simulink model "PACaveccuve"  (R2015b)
settings: Solver=ode15s  StartTime=0.0  StopTime=6000  RelTol=1e-3
libraries: fl_lib x9, nesl_utility x6

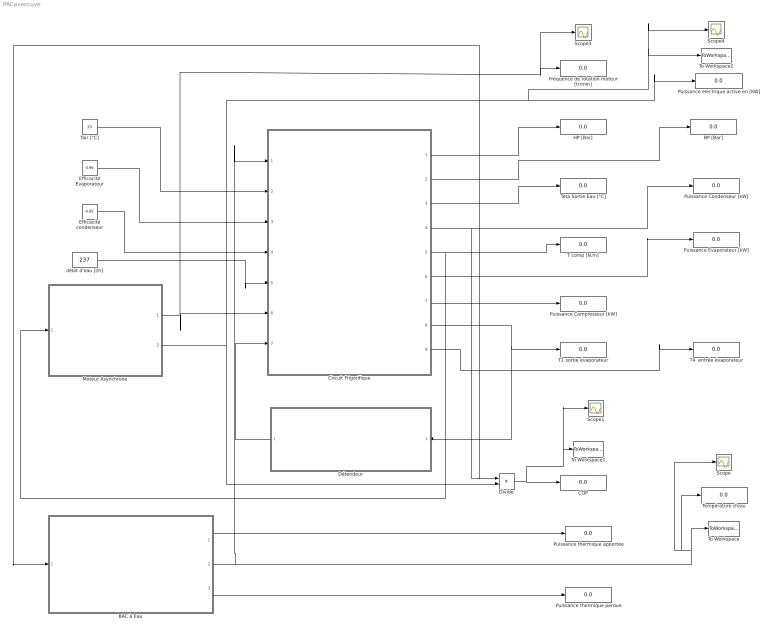
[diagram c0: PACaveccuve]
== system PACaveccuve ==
  BAC à Eau : Subsystem
  BP [Bar] : Display
  COP : Display
  Circuit Frigorifique : Subsystem
  Divide : Product  Inputs=*/
  Détendeur : Subsystem
  Efficacité Evaporateur : Constant  Value=0.99
  Efficacité condenseur : Constant  Value=0.95
  Fréquence de rotation moteur [tr/min] : Display
  HP [Bar] : Display
  Moteur Asynchrone : Subsystem
  Puissance Compresseur [kW] : Display
  Puissance Condenseur [kW] : Display
  Puissance Evaporateur [kW] : Display
  Puissance electrique active en [KW] : Display
  Puissance thermique apportée : Display
  Puissance thermique perdue : Display
  Scope{,1,3..4} (4 alike) : Scope
  T comp [N.m] : Display
  T1 sortie évaporateur : Display
  T4  entrée évaporateur : Display
  Tair [°C] : Constant  Value=23
  Température d'eau : Display
  Teta Sortie Eau [°C] : Display
  To Workspace : ToWorkspace  VariableName=Ts  SaveFormat=Timeseries  SampleTime=-1
  To Workspace1 : ToWorkspace  VariableName=COP  SaveFormat=Timeseries  SampleTime=-1
  To Workspace2 : ToWorkspace  VariableName=Pelec  SaveFormat=Timeseries  SampleTime=-1
  débit d'eau [l/h] : Constant  Value=237
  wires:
  Efficacité Evaporateur/1 -> Circuit Frigorifique/3(Eff Evapo)
  débit d'eau [l/h]/1 -> Circuit Frigorifique/5(Qv eau [l/h])
  Circuit Frigorifique/1(HP [bar]) -> HP [Bar]/1
  Circuit Frigorifique/2(BP [bar]) -> BP [Bar]/1
  Circuit Frigorifique/3(Tse [°C]) -> Teta Sortie Eau [°C]/1
  Circuit Frigorifique/5(Tm [N.m]) -> Moteur Asynchrone/1(Tm [N.m]), T comp [N.m]/1
  Circuit Frigorifique/9(T4 [°C]) -> T4  entrée évaporateur/1
  Circuit Frigorifique/8(T1 [°C]) -> Détendeur/1(T1), T1 sortie évaporateur/1
  Circuit Frigorifique/6(Pevapo [kW]) -> Puissance Evaporateur [kW]/1
  Divide/1 -> To Workspace1/1, Scope1/1, COP/1
  Circuit Frigorifique/7(Pcomp [kW]) -> Puissance Compresseur [kW]/1
  Efficacité condenseur/1 -> Circuit Frigorifique/4(effc)
  Détendeur/1(BP [Bar]) -> Circuit Frigorifique/7(BP[Bar])
  Moteur Asynchrone/2(Puissance Electrique active [W]) -> Scope4/1, To Workspace2/1, Puissance electrique active en [KW]/1, Divide/2
  Moteur Asynchrone/1(N [tr/min]) -> Scope3/1, Fréquence de rotation moteur [tr/min]/1, Circuit Frigorifique/6(N [tr/min])
  Tair [°C]/1 -> Circuit Frigorifique/2(Tair [°C])
  Circuit Frigorifique/4(Pcond [kW]) -> BAC à Eau/1(" Puissance Condenseur [kW]"), Divide/1, Puissance Condenseur [kW]/1
  BAC à Eau/2(Température du BAC [°C]) -> Scope/1, Température d'eau/1, To Workspace/1, Circuit Frigorifique/1(Tee [°C])
  BAC à Eau/1(Puissance Condenseur [W]) -> Puissance thermique apportée/1
  BAC à Eau/3(Puissance thermique perdue [W]) -> Puissance thermique perdue/1

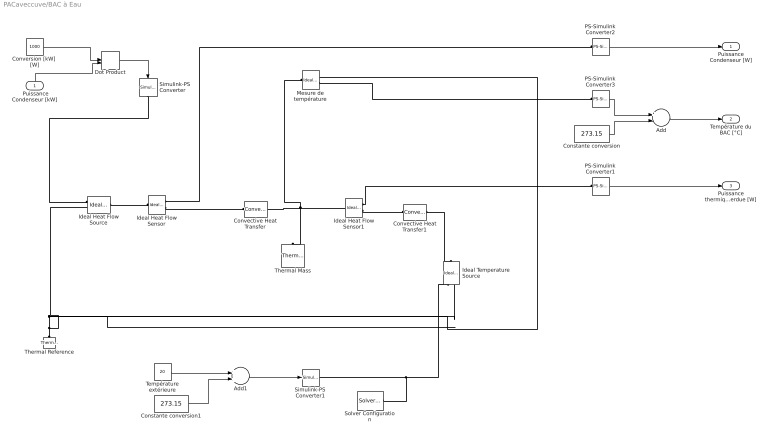
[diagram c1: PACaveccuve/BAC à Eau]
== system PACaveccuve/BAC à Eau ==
  " Puissance Condenseur [kW]" : Inport
  Add : Sum  Inputs=+-
  Add1 : Sum
  Constante conversion : Constant  Value=273.15
  Constante conversion1 : Constant  Value=273.15
  Convective Heat Transfer : fl_lib/Thermal/Thermal Elements/Convective Heat Transfer  area=1 m^2  heat_tr_coeff=1000000 W/(m^2 * K)  Q_specify=off  Q_priority=None  Q=0 J/s  T_specify=off  T_priority=None  T=0 K
  Convective Heat Transfer1 : fl_lib/Thermal/Thermal Elements/Convective Heat Transfer  area=1 m^2  heat_tr_coeff=10.3 W/(m^2 * K)  Q_specify=off  Q_priority=None  Q=0 J/s  T_specify=off  T_priority=None  T=0 K
  Conversion [kW]  [W] : Constant  Value=1000
  Dot Product : DotProduct
  Ideal Heat Flow Sensor : fl_lib/Thermal/Thermal Sensors/Ideal Heat Flow Sensor
  Ideal Heat Flow Sensor1 : fl_lib/Thermal/Thermal Sensors/Ideal Heat Flow Sensor
  Ideal Heat Flow Source : fl_lib/Thermal/Thermal Sources/Ideal Heat Flow Source
  Ideal Temperature Source : fl_lib/Thermal/Thermal Sources/Ideal Temperature Source
  Mesure de température : fl_lib/Thermal/Thermal Sensors/Ideal Temperature Sensor
  PS-Simulink Converter1 : nesl_utility/PS-Simulink Converter  PhysicalDomain=network_engine_domain  SubClassName=ps_output  LeftPortType=input  RightPortType=output  PseudoPeriodic=off  Frequencies=[]  Unit=1  AffineConversion=off
  PS-Simulink Converter2 : nesl_utility/PS-Simulink Converter  PhysicalDomain=network_engine_domain  SubClassName=ps_output  LeftPortType=input  RightPortType=output  PseudoPeriodic=off  Frequencies=[]  Unit=1  AffineConversion=off
  PS-Simulink Converter3 : nesl_utility/PS-Simulink Converter  PhysicalDomain=network_engine_domain  SubClassName=ps_output  LeftPortType=input  RightPortType=output  PseudoPeriodic=off  Frequencies=[]  Unit=1  AffineConversion=off
  Simulink-PS Converter : nesl_utility/Simulink-PS Converter  PhysicalDomain=network_engine_domain  SubClassName=ps_input  LeftPortType=input  RightPortType=output  PseudoPeriodic=off  Frequencies=[]  NoiseDistribution=none  NoiseParameters=[]  Unit=1  AffineConversion=off  InputFiltering=off  SimscapeFilterOrder=1  InputFilterTimeConstant=.001  UdotUserProvided=1
  Simulink-PS Converter1 : nesl_utility/Simulink-PS Converter  PhysicalDomain=network_engine_domain  SubClassName=ps_input  LeftPortType=input  RightPortType=output  PseudoPeriodic=off  Frequencies=[]  NoiseDistribution=none  NoiseParameters=[]  Unit=K  AffineConversion=on  InputFiltering=off  SimscapeFilterOrder=1  InputFilterTimeConstant=.001  UdotUserProvided=1
  Solver Configuration : nesl_utility/Solver Configuration  PhysicalDomain=network_engine_domain  SubClassName=solver  LeftPortType=input  RightPortType=generic  Accelerate=off  Tones=[]  Harmonics=[]  SimulateNoise=off  Profile=off  UseLocalSampling=off  EnableSwitchedLinearOptims=on  FrequencyDomain=off  UseCCode=off  RelTol=0.001  AbsTol=1e-06  MinStep=1e-09  ToWorkspace=off  RevertToSquareIcSolve=off  NumHomotopyIterations=100  PhasorMode=off  PhasorModeNumHarmonics=1  DoDC=off  ResidualTolerance=1e-9  UseLocalSolver=off  LocalSolverChoice=NE_BACKWARD_EULER_ADVANCER  LocalSolverSampleTime=.001  DoFixedCost=off  MaxNonlinIter=3  MaxModeIter=2  LinearAlgebra=Sparse  DelaysMemoryBudget=1024  AutomaticFiltering=on  FilteringTimeConstant=0.001
  Température extérieure : Constant  Value=20
  Thermal Mass : fl_lib/Thermal/Thermal Elements/Thermal Mass  mass=19.9 kg  sp_heat=4185 J/kg/K  Q_specify=off  Q_priority=None  Q=0 J/s  T_specify=on  T_priority=High  T=23.25 C
  Thermal Reference : fl_lib/Thermal/Thermal Elements/Thermal Reference
  Puissance Condenseur [W] : Outport
  Température du BAC [°C] : Outport  Port=2
  Puissance thermique perdue [W] : Outport  Port=3
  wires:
  " Puissance Condenseur [kW]"/1 -> Dot Product/2
  PS-Simulink Converter3/1 -> Add/1
  Add/1 -> Température du BAC [°C]/1
  Constante conversion/1 -> Add/2
  Dot Product/1 -> Simulink-PS Converter/1
  Conversion [kW]  [W]/1 -> Dot Product/1
  PS-Simulink Converter1/1 -> Puissance thermique perdue [W]/1
  PS-Simulink Converter2/1 -> Puissance Condenseur [W]/1
  Add1/1 -> Simulink-PS Converter1/1
  Température extérieure/1 -> Add1/1
  Constante conversion1/1 -> Add1/2
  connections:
  Thermal Reference/LConn1 -- Ideal Temperature Source/RConn2 -- Mesure de température/RConn1 -- Ideal Heat Flow Source/RConn2
  Mesure de température/LConn1 -- Thermal Mass/LConn1 -- Ideal Heat Flow Sensor1/LConn1 -- Convective Heat Transfer/RConn1
  Solver Configuration/RConn1 -- Ideal Temperature Source/RConn1 -- Simulink-PS Converter1/RConn1
  Simulink-PS Converter/RConn1 -- Ideal Heat Flow Source/RConn1
  Convective Heat Transfer1/RConn1 -- Ideal Temperature Source/LConn1
  PS-Simulink Converter3/LConn1 -- Mesure de température/RConn2
  Ideal Heat Flow Source/LConn1 -- Ideal Heat Flow Sensor/LConn1
  Ideal Heat Flow Sensor/RConn2 -- Convective Heat Transfer/LConn1
  Ideal Heat Flow Sensor1/RConn2 -- Convective Heat Transfer1/LConn1
  Ideal Heat Flow Sensor1/RConn1 -- PS-Simulink Converter1/LConn1
  Ideal Heat Flow Sensor/RConn1 -- PS-Simulink Converter2/LConn1

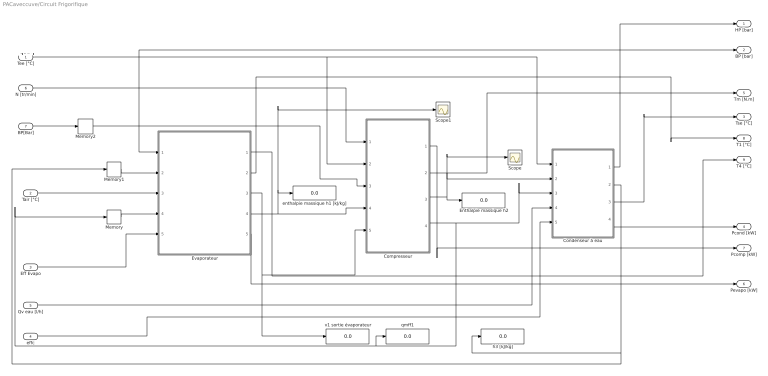
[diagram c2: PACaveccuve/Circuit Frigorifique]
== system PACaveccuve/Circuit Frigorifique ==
  note: +++++
  Tee [°C] : Inport
  Tair [°C] : Inport  Port=2
  Eff Evapo : Inport  Port=3
  effc : Inport  Port=4
  Qv eau [l/h] : Inport  Port=5
  N [tr/min] : Inport  Port=6
  BP[Bar] : Inport  Port=7
  Compresseur : Subsystem
  Condenseur à eau : Subsystem
  Enthalpie massique h2 : Display
  Evaporateur : Subsystem
  Memory : Memory  X0=0.00001
  Memory1 : Memory  X0=300
  Memory2 : Memory  X0=2.5
  Scope : Scope
  Scope1 : Scope
  enthalpie massique h1 [kJ/kg] : Display
  h3 [kJ/kg] : Display
  qmff1 : Display
  v1 sortie évaporateur : Display
  HP [bar] : Outport
  BP [bar] : Outport  Port=2
  Tse [°C] : Outport  Port=3
  Pcond [kW] : Outport  Port=4
  Tm [N.m] : Outport  Port=5
  Pevapo [kW] : Outport  Port=6
  Pcomp [kW] : Outport  Port=7
  T1 [°C] : Outport  Port=8
  T4 [°C] : Outport  Port=9
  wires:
  Evaporateur/2(T1 [°C]) -> T1 [°C]/1
  N [tr/min]/1 -> Compresseur/1(N [tr/min])
  Evaporateur/5(Pévapo [kW]) -> Pevapo [kW]/1
  Tair [°C]/1 -> Evaporateur/3(Tair [°C])
  Condenseur à eau/3(Tse [°C]) -> Tse [°C]/1
  Memory/1 -> Evaporateur/4(qmff [kg/s])
  Condenseur à eau/1(HP [bar]) -> HP [bar]/1
  BP[Bar]/1 -> Memory2/1
  Compresseur/4(qmff [kg/s]) -> Memory/1, qmff1/1, Condenseur à eau/3(qmff [kg/s])
  Tee [°C]/1 -> Compresseur/2(Tee [°C]), Condenseur à eau/1(Tee [°C])
  Eff Evapo/1 -> Evaporateur/5(Eff)
  Qv eau [l/h]/1 -> Condenseur à eau/4(qveau [l/h])
  Evaporateur/3(v1 [m3/kg]) -> v1 sortie évaporateur/1, Compresseur/5(v1 [m3/kg])
  Condenseur à eau/2(h3 [kJ/kg]) -> Memory1/1, h3 [kJ/kg]/1
  Evaporateur/4(h1 [kJ/kg]) -> Compresseur/4(h1 [kJ/kg]), Scope1/1, enthalpie massique h1 [kJ/kg]/1
  Compresseur/3(h2 [kJ/kg]) -> Scope/1, Condenseur à eau/2(h2 [kJ/kg]), Enthalpie massique h2/1
  Compresseur/2(Tm [N.m]) -> Tm [N.m]/1
  Evaporateur/1(T4 [°C]) -> T4 [°C]/1
  Condenseur à eau/4(Pcond [kW]) -> Pcond [kW]/1
  Memory1/1 -> Evaporateur/2(h3 [kJ/kg])
  Compresseur/1(Pcomp [kW]) -> Pcomp [kW]/1
  effc/1 -> Condenseur à eau/5(effc)
  Memory2/1 -> BP [bar]/1, Compresseur/3(BP [bar]), Evaporateur/1(BP [bar])

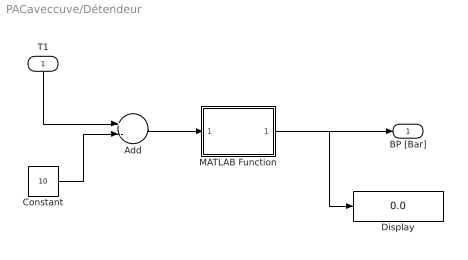
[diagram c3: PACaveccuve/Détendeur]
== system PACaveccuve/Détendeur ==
  T1 : Inport
  Add : Sum  Inputs=+-
  Constant : Constant  Value=10
  Display : Display
  MATLAB Function : MATLAB Function  TreatAsAtomicUnit=on
  BP [Bar] : Outport
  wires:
  Add/1 -> MATLAB Function/1(T)
  T1/1 -> Add/1
  Constant/1 -> Add/2
  MATLAB Function/1(BP) -> Display/1, BP [Bar]/1

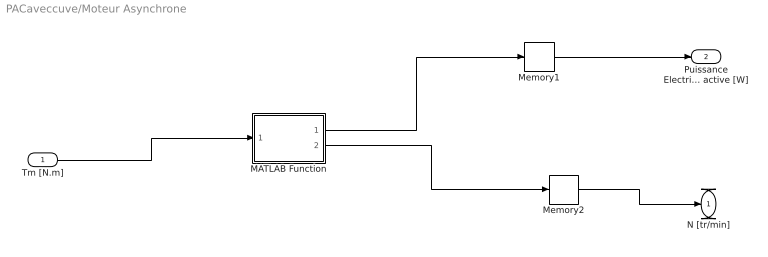
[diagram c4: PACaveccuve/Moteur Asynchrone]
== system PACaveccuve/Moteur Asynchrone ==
  Tm [N.m] : Inport
  MATLAB Function : MATLAB Function  TreatAsAtomicUnit=on
  Memory1 : Memory  X0=0.2
  Memory2 : Memory  X0=1480
  N [tr/min] : Outport
  Puissance Electrique active [W] : Outport  Port=2
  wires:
  Memory1/1 -> Puissance Electrique active [W]/1
  Memory2/1 -> N [tr/min]/1
  Tm [N.m]/1 -> MATLAB Function/1(Tm)
  MATLAB Function/1(P) -> Memory1/1
  MATLAB Function/2(N) -> Memory2/1

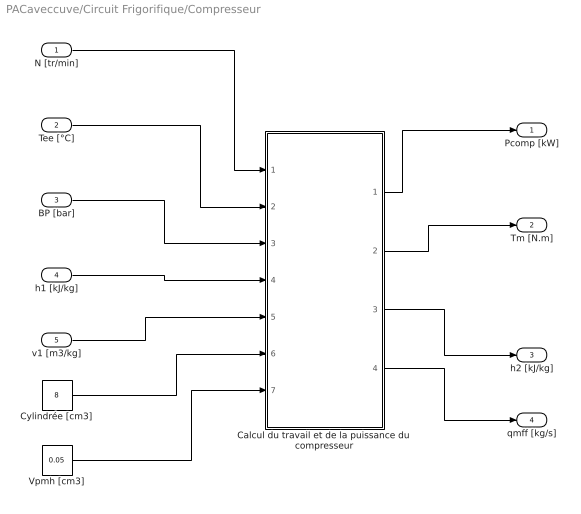
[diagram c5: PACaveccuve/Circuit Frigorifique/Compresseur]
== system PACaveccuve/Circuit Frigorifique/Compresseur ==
  N [tr/min] : Inport
  Tee [°C] : Inport  Port=2
  BP [bar] : Inport  Port=3
  h1 [kJ/kg] : Inport  Port=4
  v1 [m3/kg] : Inport  Port=5
  Calcul du travail et de la puissance du compresseur : MATLAB Function  TreatAsAtomicUnit=on
  Cylindrée [cm3] : Constant  Value=8
  Vpmh [cm3] : Constant  Value=0.05
  Pcomp [kW] : Outport
  Tm [N.m] : Outport  Port=2
  h2 [kJ/kg] : Outport  Port=3
  qmff [kg/s] : Outport  Port=4
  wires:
  Calcul du travail et de la puissance du compresseur/4(qmff) -> qmff [kg/s]/1
  Calcul du travail et de la puissance du compresseur/2(Tm) -> Tm [N.m]/1
  h1 [kJ/kg]/1 -> Calcul du travail et de la puissance du compresseur/4(h1)
  Tee [°C]/1 -> Calcul du travail et de la puissance du compresseur/2(Tee)
  BP [bar]/1 -> Calcul du travail et de la puissance du compresseur/3(BP)
  Calcul du travail et de la puissance du compresseur/1(P) -> Pcomp [kW]/1
  Calcul du travail et de la puissance du compresseur/3(h2) -> h2 [kJ/kg]/1
  N [tr/min]/1 -> Calcul du travail et de la puissance du compresseur/1(N)
  v1 [m3/kg]/1 -> Calcul du travail et de la puissance du compresseur/5(v1)
  Cylindrée [cm3]/1 -> Calcul du travail et de la puissance du compresseur/6(cyl)
  Vpmh [cm3]/1 -> Calcul du travail et de la puissance du compresseur/7(Vpmh)

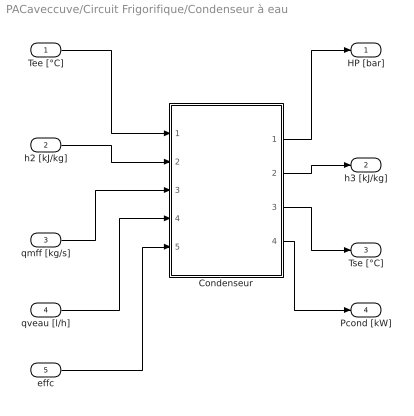
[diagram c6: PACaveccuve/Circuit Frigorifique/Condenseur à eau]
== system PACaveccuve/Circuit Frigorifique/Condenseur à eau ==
  Tee [°C] : Inport
  h2 [kJ/kg] : Inport  Port=2
  qmff [kg/s] : Inport  Port=3
  qveau [l/h] : Inport  Port=4
  effc : Inport  Port=5
  Condenseur : MATLAB Function  TreatAsAtomicUnit=on
  HP [bar] : Outport
  h3 [kJ/kg] : Outport  Port=2
  Tse [°C] : Outport  Port=3
  Pcond [kW] : Outport  Port=4
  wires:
  Tee [°C]/1 -> Condenseur/1(Tee)
  Condenseur/3(Tse) -> Tse [°C]/1
  Condenseur/1(HP) -> HP [bar]/1
  h2 [kJ/kg]/1 -> Condenseur/2(h2)
  qmff [kg/s]/1 -> Condenseur/3(qmff)
  qveau [l/h]/1 -> Condenseur/4(qveau)
  Condenseur/2(h3) -> h3 [kJ/kg]/1
  Condenseur/4(Pcond) -> Pcond [kW]/1
  effc/1 -> Condenseur/5(eff)

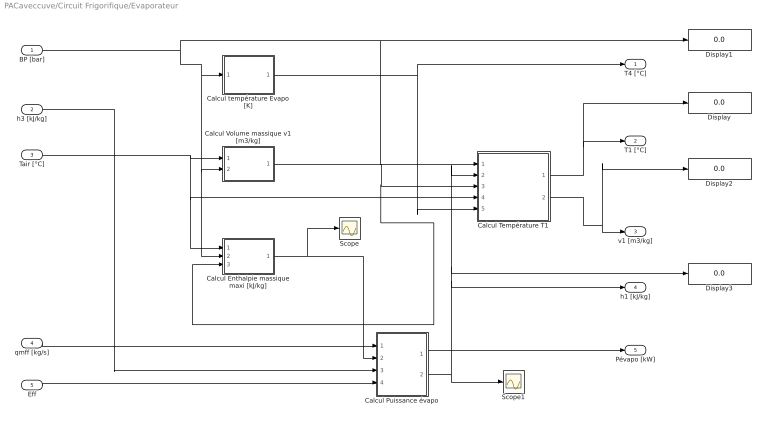
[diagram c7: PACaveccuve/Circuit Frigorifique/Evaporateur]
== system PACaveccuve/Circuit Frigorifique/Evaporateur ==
  BP [bar] : Inport
  h3 [kJ/kg] : Inport  Port=2
  Tair [°C] : Inport  Port=3
  qmff [kg/s] : Inport  Port=4
  Eff : Inport  Port=5
  Calcul Enthalpie massique maxi [kJ/kg] : MATLAB Function  TreatAsAtomicUnit=on
  Calcul Puissance évapo : MATLAB Function  TreatAsAtomicUnit=on
  Calcul Température T1 : MATLAB Function  TreatAsAtomicUnit=on
  Calcul Volume massique v1 [m3/kg] : MATLAB Function  TreatAsAtomicUnit=on
  Calcul température Evapo [K] : MATLAB Function  TreatAsAtomicUnit=on
  Display{,1..3} (4 alike) : Display
  Scope : Scope
  Scope1 : Scope
  T4 [°C] : Outport
  T1 [°C] : Outport  Port=2
  v1 [m3/kg] : Outport  Port=3
  h1 [kJ/kg] : Outport  Port=4
  Pévapo [kW] : Outport  Port=5
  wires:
  qmff [kg/s]/1 -> Calcul Puissance évapo/1(qmff)
  Calcul Enthalpie massique maxi [kJ/kg]/1(H) -> Scope/1, Calcul Puissance évapo/2(hmax)
  BP [bar]/1 -> Calcul Enthalpie massique maxi [kJ/kg]/2(P), Calcul Volume massique v1 [m3/kg]/2(P), Calcul température Evapo [K]/1(P), Display1/1, Calcul Température T1/1(P)
  Calcul température Evapo [K]/1(T) -> T4 [°C]/1, Calcul Température T1/5(T3)
  Tair [°C]/1 -> Calcul Enthalpie massique maxi [kJ/kg]/1(T), Calcul Température T1/4(T1max), Calcul Volume massique v1 [m3/kg]/1(T)
  Calcul Puissance évapo/1(Pevapo) -> Pévapo [kW]/1
  Eff/1 -> Calcul Puissance évapo/4(eff)
  Calcul Volume massique v1 [m3/kg]/1(v) -> Calcul Enthalpie massique maxi [kJ/kg]/3(v), Calcul Température T1/3(v)
  Calcul Température T1/2(v1) -> Display2/1, v1 [m3/kg]/1
  Calcul Température T1/1(T1) -> Display/1, T1 [°C]/1
  Calcul Puissance évapo/2(h1) -> h1 [kJ/kg]/1, Display3/1, Calcul Température T1/2(h), Scope1/1
  h3 [kJ/kg]/1 -> Calcul Puissance évapo/3(h3)

== matlab function PACaveccuve/Circuit Frigorifique/Compresseur/Calcul du travail
et de la puissance 
du compresseur ==
function [ P , Tm , h2 , qmff] = fcn( N , Tee , BP, h1 , v1 , cyl, Vpmh )
%#codegen

HP = 0.255 * Tee + 3.667 ;
if BP <0
BP = 1;
end
d1 = 2.49202E-01;
d2 = 2.45251E-03;
d3 = -1.65650E-06;
d4 = 8.91048E-10;
d5 = -6.96764E+00;

T = (372 + 240 )/2 ;
cp = d1 + d2 * T + d3 * T * T + d4 * T * T * T + d5 / T ;

R = 8.14892E-04 * 100;
gam = cp / (cp - R) ;

Vpmb = (cyl-Vpmh)/1000000; 
Vpmh = Vpmh/1000000;

HP = HP * 1e5;
BP = BP * 1e5;

Wtot = (HP*(BP/HP)^(1/gam)-BP)*Vpmb/(gam-1)+HP*(Vpmb*(BP/HP)^(1/gam)-Vpmh)-BP*(Vpmb-Vpmh);

if N > 0
P = Wtot * N / 60 / 1000;
else
P = 0;
end

neff = 0.85 - 0.004 * (( HP / BP - 5 ) ^2 ) - 0.5 / ( HP / BP - 0.3 );
nv = 0.9 * ( 1 + Vpmh / ( Vpmb - Vpmh ) * ( 1 - ( HP / BP ) ^ 0.72 )); 

if N > 0
qmff = nv * (Vpmb - Vpmh) / v1 * N / 60;
else
    qmff = 0;
end

h2 = h1 + Wtot /1000 / nv /(Vpmb - Vpmh) * v1 ;


Tm = Wtot / neff / 2 / 3.14 ;


end

== matlab function PACaveccuve/Circuit Frigorifique/Evaporateur/Calcul Volume massique
 v1 [m3//kg] ==
function v = f134a(T,P)
%calcule la valeur du volume spécifique à partir de T et P
T = T + 273.15 ;
%if P < 1
%    P = 1;
%end
Tc = 374.21;
%Pc = 40.59;
R = 8.14892E-04;
e1 = -1.40114E-03;
e2 = 2.19433E-06;
e3 = -6.73580E-10;
e4 = -4.66800E-12;
f1 = 1.63714E-06;
f2 = -2.78860E-09;
f4 = 1.02574E-14;
g1 = -2.69555E-02;
g2 = 2.67772E-05;
g4 = 1.69513E-10;

b = 2.99628E-04;
k = 5.475;

Tr = T / Tc;
Zmax = 1;
Zmin = 0.008;
z = 0;    
    while Zmax - Zmin >= 0.00000001
    Zmoy = (Zmax + Zmin) / 2;
    z = Zmoy;
    zer = P - R * T / z - (e1 + f1 * T + g1 * exp(-k * Tr)) / (z * z) - (e2 + f2 * T + g2 * exp(-k * Tr)) / (z * z * z) - e3 / (z * z * z * z) - (e4 + f4 * T + g4 * exp(-k * Tr)) / (z * z * z * z * z);
    fzmoy = zer;
    z = Zmin;
    zer = P - R * T / z - (e1 + f1 * T + g1 * exp(-k * Tr)) / (z * z) - (e2 + f2 * T + g2 * exp(-k * Tr)) / (z * z * z) - e3 / (z * z * z * z) - (e4 + f4 * T + g4 * exp(-k * Tr)) / (z * z * z * z * z);
    fzmin = zer;

        if fzmoy * fzmin < 0
        Zmax = Zmoy;
        elseif fzmoy * fzmin > 0
        Zmin = Zmoy;
        end
        z = Zmoy;
        
    end
        
    v = z + b ;
    
end

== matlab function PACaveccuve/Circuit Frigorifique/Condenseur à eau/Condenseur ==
function [HP, h3 ,Tse, Pcond] = fcn(Tee,h2,qmff,qveau,eff)
%#codegen
Tc = 374.21;

HP = 0,002*Tee^2 + 0,067*Tee + 8,841; %0.232 * Tee + 5.497 ;

Tr = (Tee + 273.15)/Tc;

h3max = 13807 * Tr ^5 - 50330* Tr^4 + 73272 * Tr^3 - 53050 * Tr ^2 + 19531* Tr - 2860;

h3 = h2 - (h2 - h3max)* eff;
if qmff >0
Pcond  = (h2 -h3)*qmff ;
else
   Pcond = 0;
end   
Tse = Tee + (Pcond )*1000 / 4185 / ( qveau / 3600);

end

== matlab function PACaveccuve/Circuit Frigorifique/Evaporateur/Calcul température Evapo
[K] ==
function T = f134a(P)
% calcul de la BP à partir de la valeur de la température
if P < 1
    P = 1;
end
a1g = -7.7069E+00;
a2g = 2.4932E+00;
a3g = -2.9212E+00;
a4g = -3.8684E+00;
a5g = 4.6898E-01;
a6g = -8.3360E-05;
b1 = 1.5158;
b2 = 1.9907;
b3 = 4.3798;
b4 = 1.7461;
Tc = 374.21;
Pc = 40.59; 
Pr = P / Pc;

Tmax = Tc;
Tmin = 100;
Tmoy = 100;
while Tmax - Tmin >= 0.000000001
Tmoy = (Tmax + Tmin) / 2 ;
Tr = Tmoy / Tc;
zer = Pr - exp((a1g * (1 - Tr) + a2g * (1 - Tr) ^ b1 + a3g * (1 - Tr) ^ b2 + a4g * (1 - Tr) ^ b3 + a5g * (1 - Tr) ^ b4 + a6g) / Tr);
zermax = zer;
Tr = Tmin / Tc;
zer = Pr - exp((a1g * (1 - Tr) + a2g * (1 - Tr) ^ b1 + a3g * (1 - Tr) ^ b2 + a4g * (1 - Tr) ^ b3 + a5g * (1 - Tr) ^ b4 + a6g) / Tr);
zermin = zer;

if zermax * zermin < 0
    Tmax = Tmoy ;
elseif zermax * zermin > 0
    Tmin = Tmoy ;
end
Tmoy = (Tmax + Tmin) / 2 ;

end
    
       
T = Tmoy-273.15; %Tr * Tc;
end

== matlab function PACaveccuve/Circuit Frigorifique/Evaporateur/Calcul Enthalpie massique
 maxi [kJ//kg] ==
function H = f134a(T,P,v)
%calcule la valeur du volume spécifique à partir de T et P



Tc = 374.21;
Pc = 40.59;

R = 8.14892E-04;

d1 = 2.49202E-01;
d2 = 2.45251E-03;
d3 = -1.65650E-06;
%d4 = 8.91048E-10;
d5 = -6.96764E+00;

e1 = -1.40114E-03;
e2 = 2.19433E-06;
e3 = -6.73580E-10;
e4 = -4.66800E-12;

%f1 = 1.63714E-06;
%f2 = -2.78860E-09;
%f4 = 1.02574E-14;

g1 = -2.69555E-02;
g2 = 2.67772E-05;
g4 = 1.69513E-10;

b = 2.99628E-04;
k = 5.475;

Ho = 295.57 ;

z = v - b;
T = T + 273.15;
Tr = T / Tc ;

H = Ho + 100*(P * v - R * T) + d1 * T + d2 * T * T /2 + d3 * T * T * T / 3 + d5 * log(T) + 100* ( e1 / z + e2 / 2 / z / z + e3 / 3 / z / z / z + e4 / 4 / z / z / z / z + exp(-k*Tr)*(1+k*Tr) * ( g1 / z + g2 / 2 / z / z + g4 / 4 / z / z / z / z ));


    
end

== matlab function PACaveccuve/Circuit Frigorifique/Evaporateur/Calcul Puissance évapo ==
function [Pevapo,h1] = f134a(qmff,hmax,h3,eff)
%calcule la valeur du volume spécifique à partir de T et P
h1 = h3 + (hmax - h3 ) * eff ;
Pevapo = qmff * (hmax -h3) * eff;
    
end

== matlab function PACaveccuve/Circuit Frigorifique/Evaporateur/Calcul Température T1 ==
function [T1,v1] = f134a(P,h,v,T1max,T3)
%calcule la valeur du volume spécifique à partir de T et P

T1max = T1max + 273.15;
T3 = T3 + 273.15;
if P < 1
    P = 1;
end

R = 8.14892E-04;
Tc = 374.21;
Pc = 40.59;
d1 = 2.49202E-01;
d2 = 2.45251E-03;
d3 = -1.65650E-06;
%d4 = 8.91048E-10;
d5 = -6.96764E+00;

e1 = -1.40114E-03;
e2 = 2.19433E-06;
e3 = -6.73580E-10;
e4 = -4.66800E-12;

f1 = 1.63714E-06;
f2 = -2.78860E-09;
f4 = 1.02574E-14;

g1 = -2.69555E-02;
g2 = 2.67772E-05;
g4 = 1.69513E-10;

b = 2.99628E-04;
k = 5.475;

Ho = 295.57 ;

Tmax = T1max;
Tmin = T3 ;
T = 0;

while (Tmax - Tmin) >= 0.001
    
Tmoy = ( Tmax + Tmin ) / 2 ;

T = Tmoy;
Tr = T / Tc ;

Zmax = 1;
Zmin = 0.008;
z = 0;    
    while Zmax - Zmin >= 0.00000001
    Zmoy = (Zmax + Zmin) / 2;
    z = Zmoy;
    zer = P - R * T / z - (e1 + f1 * T + g1 * exp(-k * Tr)) / (z * z) - (e2 + f2 * T + g2 * exp(-k * Tr)) / (z * z * z) - e3 / (z * z * z * z) - (e4 + f4 * T + g4 * exp(-k * Tr)) / (z * z * z * z * z);
    fzmoy = zer;
    z = Zmin;
    zer = P - R * T / z - (e1 + f1 * T + g1 * exp(-k * Tr)) / (z * z) - (e2 + f2 * T + g2 * exp(-k * Tr)) / (z * z * z) - e3 / (z * z * z * z) - (e4 + f4 * T + g4 * exp(-k * Tr)) / (z * z * z * z * z);
    fzmin = zer;

        if fzmoy * fzmin < 0
        Zmax = Zmoy;
        elseif fzmoy * fzmin > 0
        Zmin = Zmoy;
        end
        z = Zmoy;
        
    end
        
    v = z + b ;
    
zerhmax = h - (Ho + 100*(P * v - R * T) + d1 * T + d2 * T * T /2 + d3 * T * T * T / 3 + d5 * log(T) + 100* ( e1 / z + e2 / 2 / z / z + e3 / 3 / z / z / z + e4 / 4 / z / z / z / z + exp(-k*Tr)*(1+k*Tr) * ( g1 / z + g2 / 2 / z / z + g4 / 4 / z / z / z / z )));

T = Tmin;
Tr = T / Tc ;

Zmax = 1;
Zmin = 0.008;
z = 0;    
    while Zmax - Zmin >= 0.00000001
    Zmoy = (Zmax + Zmin) / 2;
    z = Zmoy;
    zer = P - R * T / z - (e1 + f1 * T + g1 * exp(-k * Tr)) / (z * z) - (e2 + f2 * T + g2 * exp(-k * Tr)) / (z * z * z) - e3 / (z * z * z * z) - (e4 + f4 * T + g4 * exp(-k * Tr)) / (z * z * z * z * z);
    fzmoy = zer;
    z = Zmin;
    zer = P - R * T / z - (e1 + f1 * T + g1 * exp(-k * Tr)) / (z * z) - (e2 + f2 * T + g2 * exp(-k * Tr)) / (z * z * z) - e3 / (z * z * z * z) - (e4 + f4 * T + g4 * exp(-k * Tr)) / (z * z * z * z * z);
    fzmin = zer;

        if fzmoy * fzmin < 0
        Zmax = Zmoy;
        elseif fzmoy * fzmin > 0
        Zmin = Zmoy;
        end
        z = Zmoy;
        
    end
        
    v = z + b ;

zerhmin = h - (Ho + 100*(P * v - R * T) + d1 * T + d2 * T * T /2 + d3 * T * T * T / 3 + d5 * log(T) + 100* ( e1 / z + e2 / 2 / z / z + e3 / 3 / z / z / z + e4 / 4 / z / z / z / z + exp(-k*Tr)*(1+k*Tr) * ( g1 / z + g2 / 2 / z / z + g4 / 4 / z / z / z / z )));


     if zerhmax*zerhmin < 0
        Tmax = Tmoy;
        elseif zerhmax*zerhmin > 0
        Tmin = Tmoy;
     end
        
end
   T1 = T-273.15;
   v1 = v;
end

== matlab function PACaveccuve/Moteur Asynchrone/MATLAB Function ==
function [P,N] = fcn(Tm)
%#codegen
N = 1496 - 12.95*Tm ;
P = (Tm * N / 60 * 2 * 3.14 / (0.004511*Tm^5 - 0.0626*Tm^4 + 0.3357*Tm^3-0.905*Tm^2+1.0198*Tm +0.12 ) )/1000 ;% (0.004511*Tm^5 - 0.0626*Tm^4 + 0.3357*Tm^3-0.905*Tm^2+1.0198*Tm +0.02)(0.003*Tm^5 - 0.045*Tm^4 + 0.228*Tm^3 - 0.553*Tm^2 + 0.779*Tm + 0.02))/1000 ;
end

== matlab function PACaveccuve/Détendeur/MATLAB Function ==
function BP = f134a(T)
% calcul de la BP à partir de la valeur de la température
T= T + 273.15;
a1g = -7.7069E+00;
a2g = 2.4932E+00;
a3g = -2.9212E+00;
a4g = -3.8684E+00;
a5g = 4.6898E-01;
a6g = -8.3360E-05;
b1 = 1.5158;
b2 = 1.9907;
b3 = 4.3798;
b4 = 1.7461;
Tc = 374.21;
Pc = 40.59; 
Tr = T / Tc;
Pr = exp((a1g * (1 - Tr) + a2g * (1 - Tr) ^ b1 + a3g * (1 - Tr) ^ b2 + a4g * (1 - Tr) ^ b3 + a5g * (1 - Tr) ^ b4 + a6g) / Tr);
BP = Pr * Pc;


end
